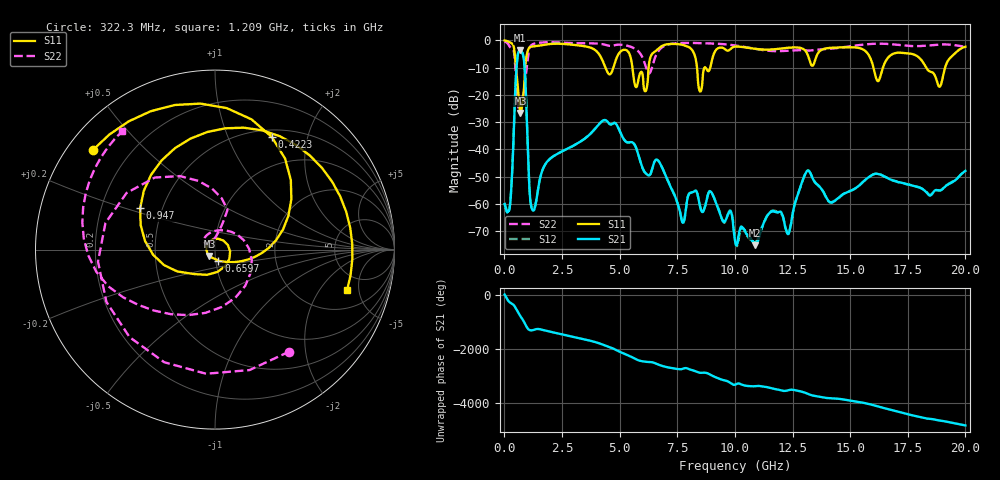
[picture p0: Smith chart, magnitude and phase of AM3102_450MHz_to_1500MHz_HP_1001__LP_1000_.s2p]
!Agilent Technologies,E8364B,MY43040894,A.07.50.67
!Agilent E8364B: A.07.50.67
!Date: Thursday, January 11, 2018 06:03:23
!Correction: S11(Full 2 Port(1,2))
!S21(Full 2 Port(1,2))
!S12(Full 2 Port(1,2))
!S22(Full 2 Port(1,2))
!S2P File: Measurements: S11, S21, S12, S22:
# Hz S  dB  R 50
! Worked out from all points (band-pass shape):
!   1601 points, 10 MHz to 20 GHz, reference 50 ohm
!   highest |S21| = -3.69 dB at 672.2 MHz (marker M1); lowest = -75.3 dB at 10.88 GHz (marker M2)
!   |S21| within 3 dB of the highest: 561.3 MHz to 840.4 MHz (279 MHz wide, 39.8 % of centre)
!   lowest |S11| = -26.6 dB at 697.2 MHz (marker M3), VSWR 1.10, Z = 46.9 - j3.3 ohm
!   |S11| at or under -10 dB: 5.555 GHz to 6.256 GHz (701 MHz wide, 11.9 % of centre); 16.01 GHz to 16.42 GHz (412.2 MHz wide, 2.54 % of centre); 18.3 GHz to 19.12 GHz (822.1 MHz wide, 4.39 % of centre)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
!   |S22| runs from -26.0 to -0.4 dB; largest |S21 - S12| = 0.00097
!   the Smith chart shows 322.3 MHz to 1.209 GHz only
!   S11 on the Smith chart (normalised r, x): 322.3 MHz: 0.07, +0.35; 422.3 MHz: 0.59, +1.46; 659.7 MHz: 1.03, -0.13; 947 MHz: 0.37, +0.23; 1.209 GHz: 3.38, -3.74
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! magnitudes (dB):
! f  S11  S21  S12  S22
! 10 MHz  -0.1  -60.1  -59.7  -0.4
! 322.3 MHz  -1.1  -51.0  -50.8  -3.1
! 422.3 MHz  -3.1  -29.2  -29.3  -4.7
! 659.7 MHz  -23.8  -3.7  -3.7  -25.9
! 672.2 MHz  -25.5  -3.7  -3.7  -25.9
! 697.2 MHz  -26.6  -3.7  -3.7  -25.4
! 947 MHz  -6.4  -22.6  -22.6  -11.6
! 1.209 GHz  -2.3  -62.2  -61.6  -1.5
! 3.346 GHz  -2.0  -36.9  -36.9  -1.1
! 4.795 GHz  -8.2  -30.3  -30.3  -1.8
! 6.119 GHz  -18.7  -48.7  -48.8  -9.2
! 6.682 GHz  -3.0  -44.2  -44.2  -3.9
! 7.731 GHz  -1.7  -66.9  -67.0  -1.0
! 8.493 GHz  -18.8  -61.0  -61.2  -1.0
! 10.01 GHz  -2.3  -73.5  -73.2  -1.9
! 10.88 GHz  -3.1  -75.3  -74.2  -3.1
! 11.6 GHz  -3.4  -62.7  -62.6  -3.9
! 12.33 GHz  -2.7  -71.1  -70.7  -3.8
! 13.34 GHz  -9.3  -50.0  -49.9  -3.7
! 16.68 GHz  -6.1  -50.8  -50.7  -1.4
! 18.88 GHz  -17.1  -55.1  -55.1  -1.6
! 20 GHz  -2.4  -47.9  -47.8  -2.3
